FUNCTION_BLOCK FB_ProxyPLCCalculationTcComModule EXTENDS FB_ProxyPLCTcComModule
VAR_INPUT
END_VAR
VAR_OUTPUT
END_VAR
VAR
	_iThisProvider		: I_Calculation;
END_VAR

METHOD AfterProviderInit : BOOL
VAR_INPUT
	IID				: IID;
END_VAR


SUPER^.AfterProviderInit(IID:= IID	);

ComQueryInterface(Super^._iProvider,TC_GLOBAL_IID_LIST.IID_I_Calculation ,ADR(_iThisProvider));
END_METHOD

PROPERTY ip : I_Calculation
GET
ip	:= _iThisProvider;
END_GET
END_PROPERTY

END_FUNCTION_BLOCK
